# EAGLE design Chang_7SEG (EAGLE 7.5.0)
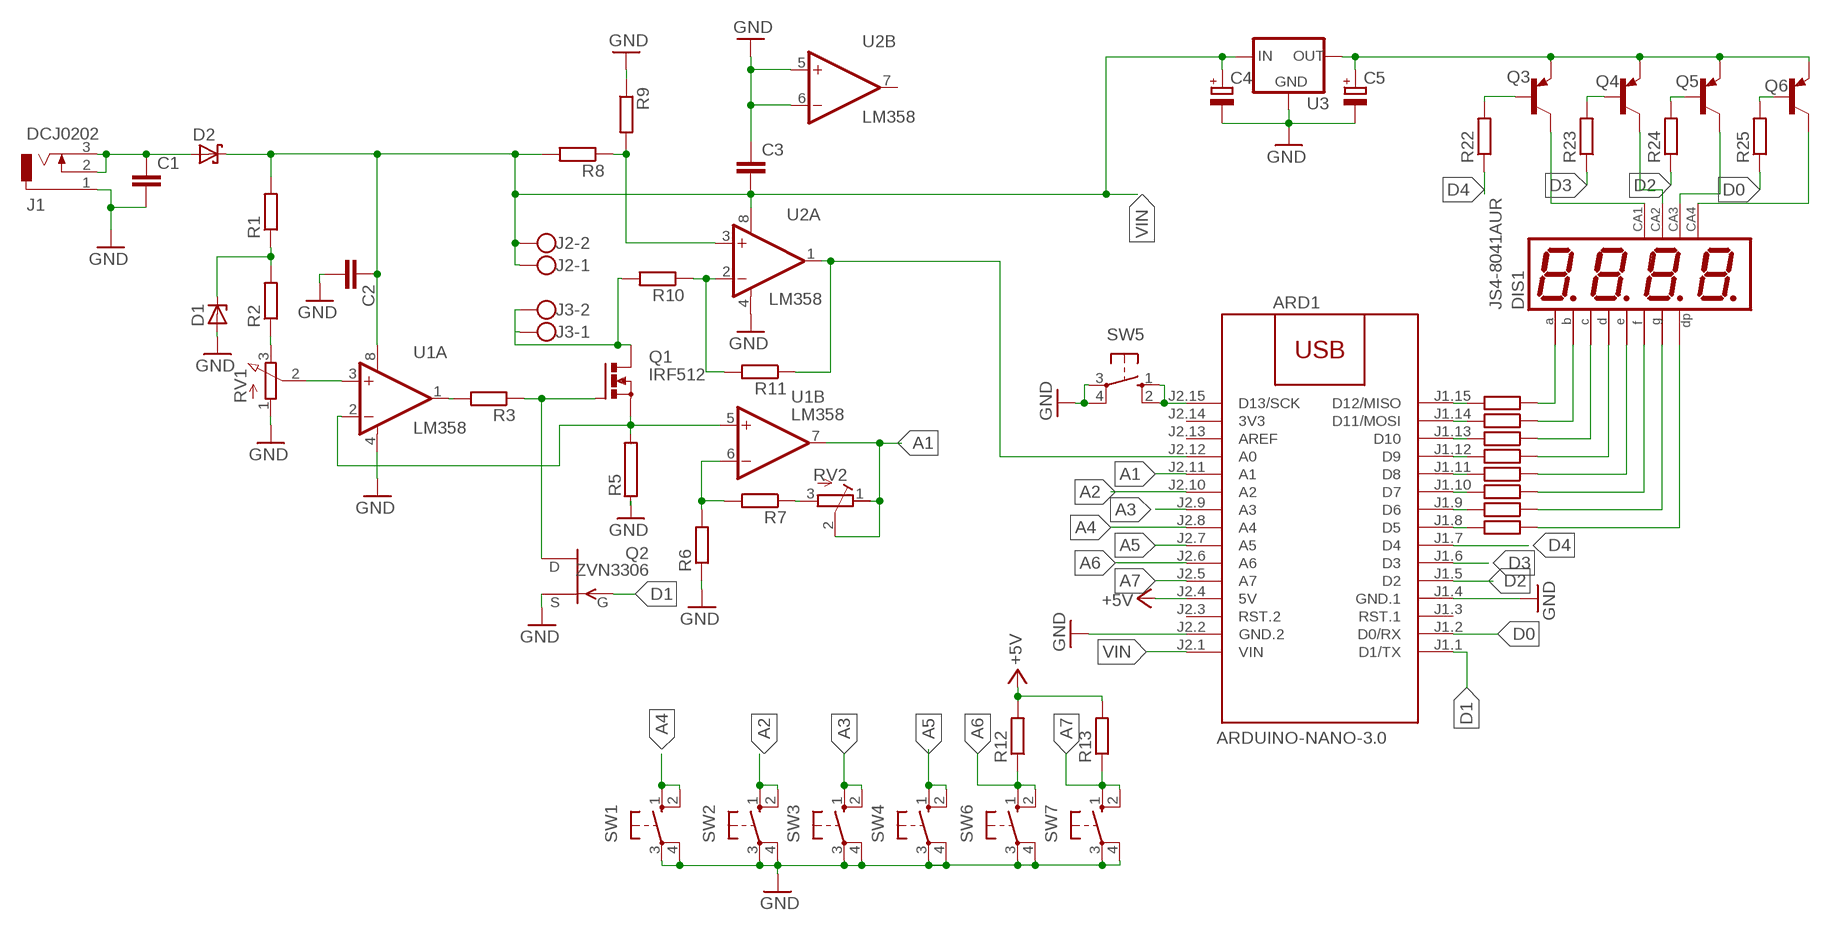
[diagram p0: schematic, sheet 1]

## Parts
ARD1  ARDUINO-NANO-3.0  [ARDUINO-NANO-3.0]
C1  C-EUC1206  [C1206]
C2  C-EUC1206  [C1206]
C3  C-EUC1206  [C1206]
C4  CPOL-EUSMCC  [SMC_C]
C5  CPOL-EUSMCC  [SMC_C]
D1  1N4728  [DO41Z10]
D2  MBR1560  [TO220ACS]
DIS1  JS4-8041AUR  [0.8INCH-4DIG]
J1  DCJ0202  [DCJ0202]
J2  W237-102  [W237-102]
J3  W237-102  [W237-102]
Q1  IRF512  [TO220BV]
Q2  ZVN3306  2N3819  [TO92]
Q3  BC328  [TO92-EBC]
Q4  BC328  [TO92-EBC]
Q5  BC328  [TO92-EBC]
Q6  BC328  [TO92-EBC]
R1  R-EU_R1206  [R1206]
R2  R-EU_R1206  [R1206]
R3  R-EU_R1206  [R1206]
R5  RAC04  [AC04]
R6  R-EU_R1206  [R1206]
R7  R-EU_R1206  [R1206]
R8  R-EU_R1206  [R1206]
R9  R-EU_R1206  [R1206]
R10  R-EU_R1206  [R1206]
R11  R-EU_R1206  [R1206]
R12  R-EU_R1206  [R1206]
R13  R-EU_R1206  [R1206]
R14  R-EU_R1206  [R1206]
R15  R-EU_R1206  [R1206]
R16  R-EU_R1206  [R1206]
R17  R-EU_R1206  [R1206]
R18  R-EU_R1206  [R1206]
R19  R-EU_R1206  [R1206]
R20  R-EU_R1206  [R1206]
R21  R-EU_R1206  [R1206]
R22  R-EU_R1206  [R1206]
R23  R-EU_R1206  [R1206]
R24  R-EU_R1206  [R1206]
R25  R-EU_R1206  [R1206]
RV1  PV09A  [PTV09]
RV2  R-TRIMM-3386-F  [R-TRIMM-3386F]
SW1  40-XX  [B3F-40XX]
SW2  40-XX  [B3F-40XX]
SW3  40-XX  [B3F-40XX]
SW4  40-XX  [B3F-40XX]
SW5  40-XX  [B3F-40XX]
SW6  40-XX  [B3F-40XX]
SW7  40-XX  [B3F-40XX]
U1  LM358  OPA2650P  [DIL08]
U2  LM358  OPA2650P  [DIL08]
U3  78XXS  [78XXS]

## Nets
+5V: ARD1.J2.4(5V) R12.2 R13.2
A1: ARD1.J2.11(A1) RV2.1(A) RV2.2(S) U1.7(B:OUT)
A2: ARD1.J2.10(A2) SW2.1(S) SW2.2(S1)
A3: ARD1.J2.9(A3) SW3.1(S) SW3.2(S1)
A4: ARD1.J2.8(A4) SW1.1(S) SW1.2(S1)
A5: ARD1.J2.7(A5) SW4.1(S) SW4.2(S1)
A6: ARD1.J2.6(A6) R12.1 SW6.1(S) SW6.2(S1)
A7: ARD1.J2.5(A7) R13.1 SW7.1(S) SW7.2(S1)
D0: ARD1.J1.2(D0/RX) R25.1
D1: ARD1.J1.1(D1/TX) Q2.2(G)
D2: ARD1.J1.5(D2) R24.1
D3: ARD1.J1.6(D3) R23.1
D4: ARD1.J1.7(D4) R22.1
GND: ARD1.J1.4(GND.1) ARD1.J2.2(GND.2) C1.2 C2.2 C3.1 C4.- C5.- D1.A J1.1 Q2.3(S) R5.1 R6.1 R9.1 RV1.1(A) SW1.3(P) SW1.4(P1) SW2.3(P) SW2.4(P1) SW3.3(P) SW3.4(P1) SW4.3(P) SW4.4(P1) SW5.3(P) SW5.4(P1) SW6.3(P) SW6.4(P1) SW7.3(P) SW7.4(P1) U1.4(A:V-) U2.4(A:V-) U2.5(B:+IN) U2.6(B:-IN) U3.GND
N$1: Q3.B R22.2
N$2: Q4.B R23.2
N$3: DIS1.12(CA) Q3.C
N$4: DIS1.9(CA) Q4.C
N$5: Q5.B R24.2
N$6: DIS1.8(CA) Q5.C
N$7: C1.1 D2.A J1.2 J1.3
N$8: Q6.B R25.2
N$9: DIS1.6(CA4) Q6.C
N$10: ARD1.J1.15(D12/MISO) R14.2
N$11: ARD1.J1.14(D11/MOSI) R15.2
N$12: ARD1.J1.13(D10) R16.2
N$13: ARD1.J1.12(D9) R17.2
N$14: ARD1.J1.11(D8) R18.2
N$15: ARD1.J1.10(D7) R19.2
N$16: ARD1.J1.9(D6) R20.2
N$17: ARD1.J1.8(D5) R21.2
N$18: DIS1.11(A) R14.1
N$19: DIS1.7(B) R15.1
N$20: DIS1.4(C) R16.1
N$21: DIS1.2(D) R17.1
N$22: DIS1.1(E) R18.1
N$23: DIS1.10(F) R19.1
N$24: DIS1.5(G) R20.1
N$25: DIS1.3(DP) R21.1
N$26: C5.+ Q3.E Q4.E Q5.E Q6.E U3.OUT
N$27: R2.1 RV1.3(E)
N$28: RV1.2(S) U1.3(A:+IN)
N$29: D1.C R1.1 R2.2
N$30: R3.2 U1.1(A:OUT)
N$31: ARD1.J2.15(D13/SCK) SW5.1(S) SW5.2(S1)
N$32: Q1.G Q2.1(D) R3.1
N$33: Q1.S R5.2 U1.2(A:-IN) U1.5(B:+IN)
N$34: J3.1 J3.2 Q1.D R10.2
N$35: R7.1 RV2.3(E)
N$36: R6.2 R7.2 U1.6(B:-IN)
N$37: R8.1 R9.2 U2.3(A:+IN)
N$38: R10.1 R11.2 U2.2(A:-IN)
N$39: ARD1.J2.12(A0) R11.1 U2.1(A:OUT)
VIN: ARD1.J2.1(VIN) C2.1 C3.2 C4.+ D2.C J2.1 J2.2 R1.2 R8.2 U1.8(A:V+) U2.8(A:V+) U3.IN
Unconnected: ARD1.J1.3(RST.1) ARD1.J2.3(RST.2) ARD1.J2.13(AREF) U2.7(B:OUT)

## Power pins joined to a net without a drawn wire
3V3: ARD1.J2.14(3V3)

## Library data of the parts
ARD1 = diy-modules:ARDUINO-NANO-3.0: Arduino Nano 3.0 and compatible devices More details available here: https://www.arduino.cc/en/Main/ArduinoBoardNano Click here to find device on ebay.com
C1-C3 = rcl:C-EU: CAPACITOR, European symbol
C4 C5 = rcl:CPOL-EU: POLARIZED CAPACITOR, European symbol
D1 = diode:1N4728: Z DIODE
D2 = diode:MBR1560
DIS1 = display-kingbright:JS4-8041AUR: 0.8in 4digit display CA
J1 = con-jack:DCJ0202: DC POWER JACK Source: DCJ0202.pdf; OC_FARNELL: unknown; OC_NEWARK: unknown
J2 J3 = con-wago-500:W237-102: WAGO SCREW CLAMP; MPN: 237-102; OC_FARNELL: unknown; OC_NEWARK: 70K9898
Q1 = transistor-power:IRF512: N-CHANNEL MOS FET
Q2 = transistor-fet:2N3819: N-Channel Junction FET
Q3-Q6 = transistor-pnp:BC328*: PNP Transistror
R1-R3 R6-R25 = rcl:R-EU_: RESISTOR, European symbol
R5 = resistor-power:R: Power Resitor; OC_FARNELL: unknown; OC_NEWARK: unknown
RV1 = pot:PV09A
RV2 = rcl:R-TRIMM-3386-F
SW1-SW7 = switch-omron:40-XX: OMRON SWITCH; MF: OMRON COMPONENTS USA; MPN: B3F-4000; OC_FARNELL: 176434; OC_NEWARK: 36K3105
U1 U2 = burr-brown:OPA2650: Dual Wideband, Low Power Voltage Feedback Operational Amplifier; MPN: AD8056ANZ; OC_FARNELL: 1079308; OC_NEWARK: 19M0925
U3 = v-reg:78XXS: VOLTAGE REGULATOR

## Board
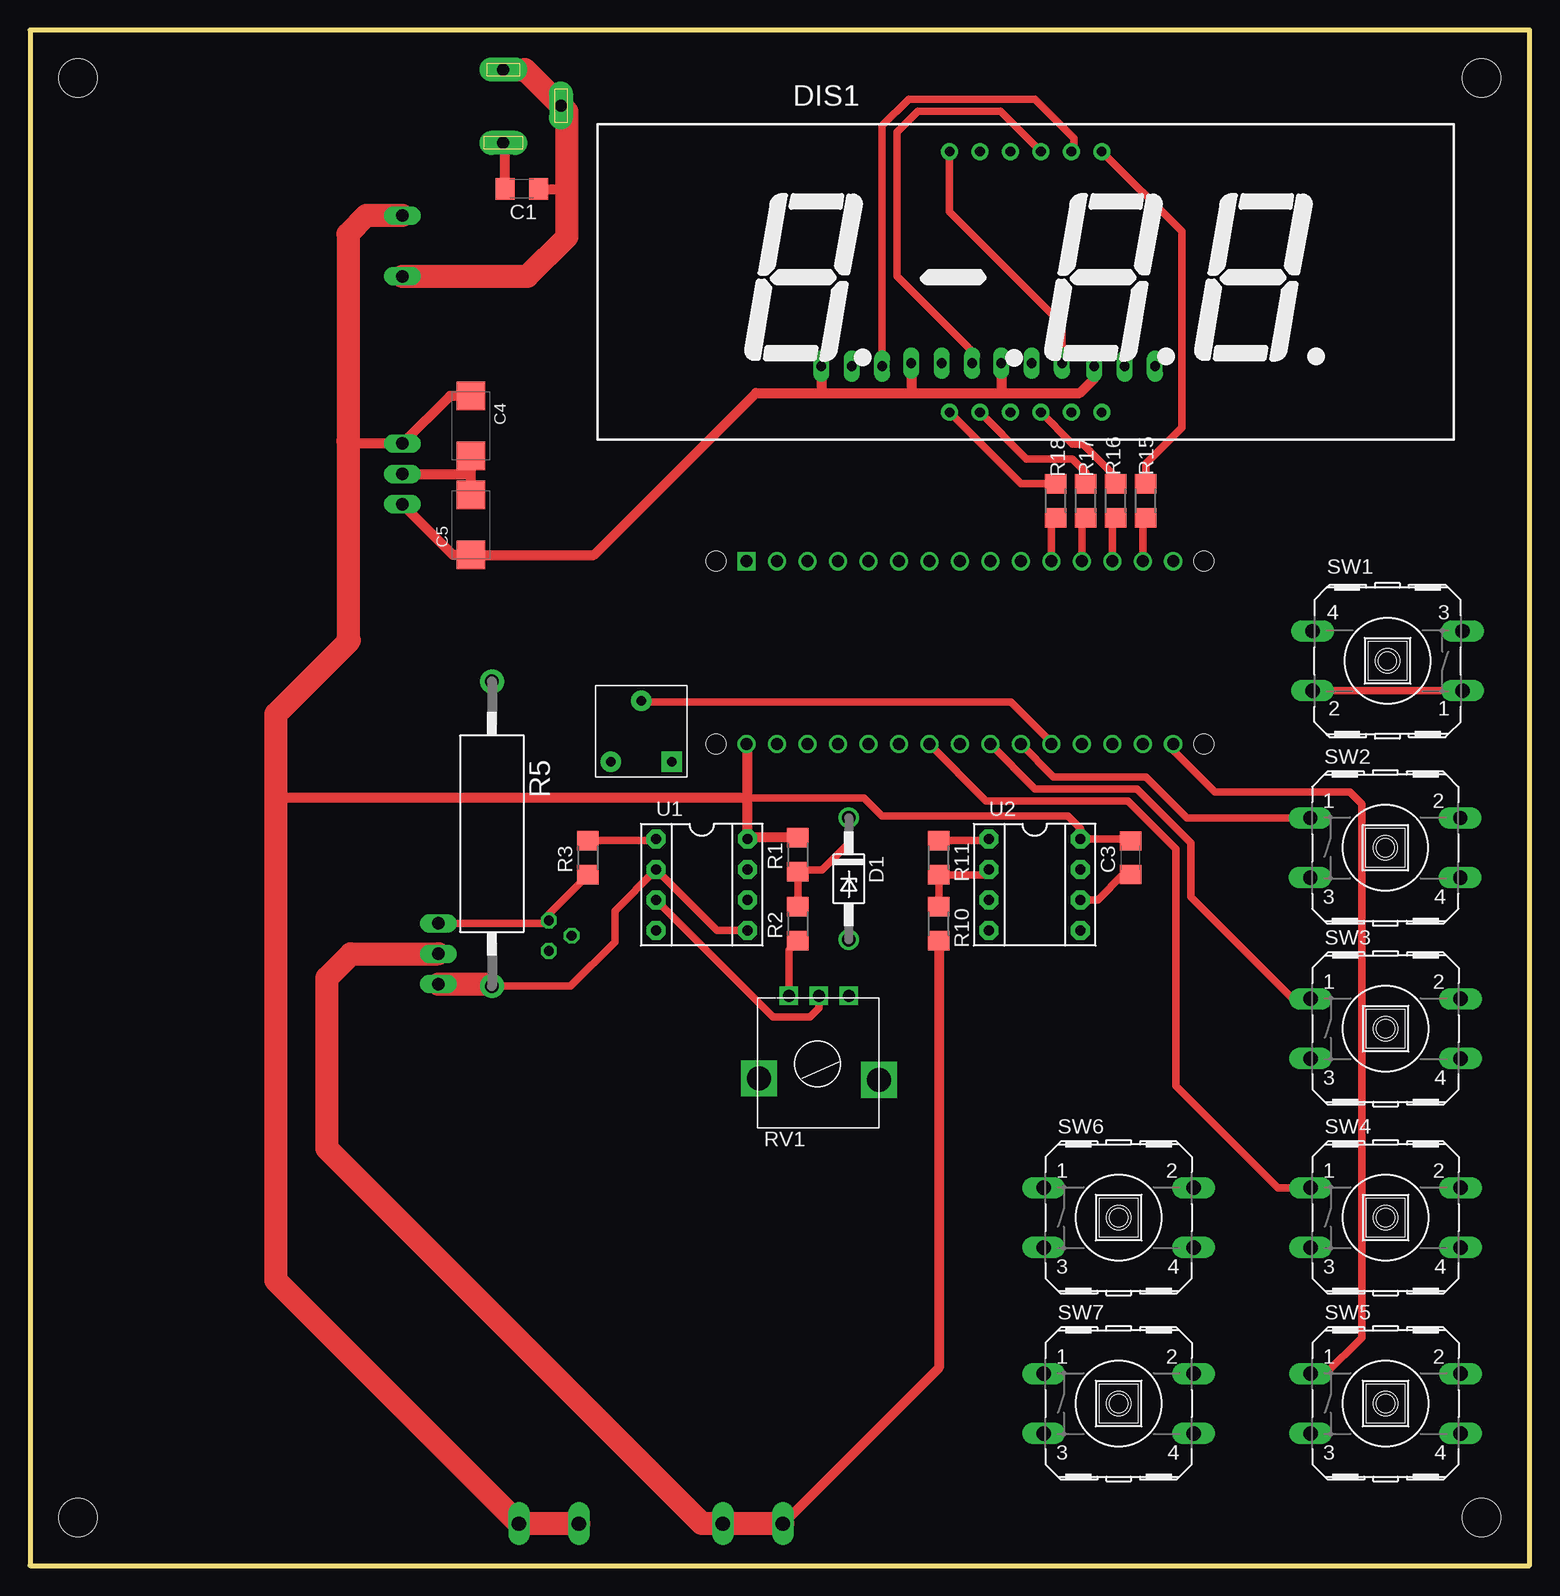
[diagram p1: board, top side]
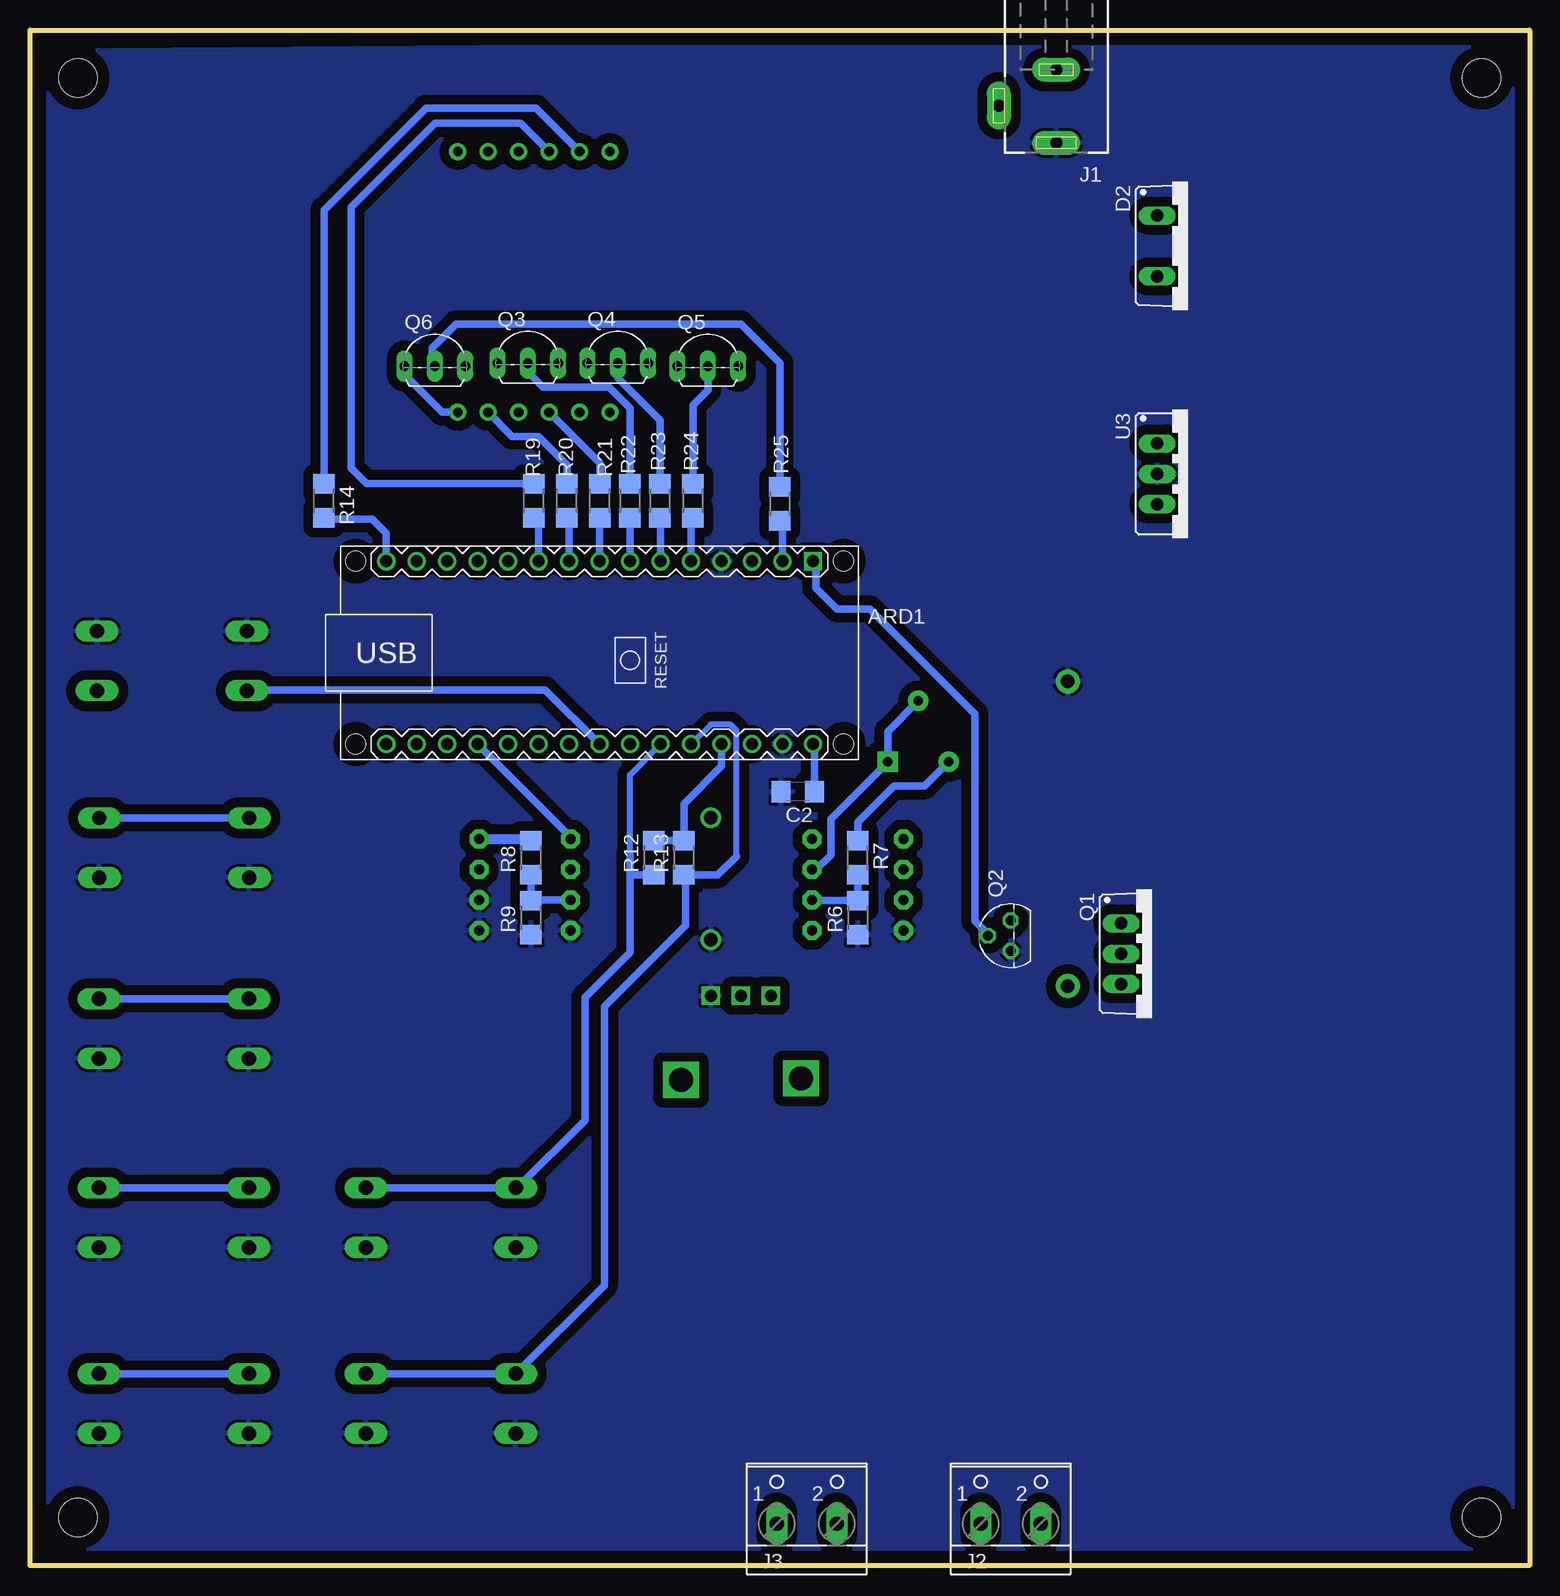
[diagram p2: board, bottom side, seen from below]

Size 125 x 128 mm. Coordinates in mm from the lower left corner, seen from the top.
Outline: 0,0 125,0 125,128 0,128 0,0
Copper layers (1*16): Top 0.035mm / dielectric 1.5mm / Bottom 0.035mm
Design rules "default": minimum track width 10mil, minimum drill 24mil, track to track 8mil, track to pad 8mil, pad to pad 8mil, via to via 8mil, smd to smd 8mil, copper to edge 40mil, drill to drill 8mil, minimum pad ring 10mil, minimum via ring 8mil, stop-mask expansion 4mil, vias tented up to drill 0mil, thermal gap 10mil
Holes 3.2 mm at 4,4 121,4 4,124 121,124

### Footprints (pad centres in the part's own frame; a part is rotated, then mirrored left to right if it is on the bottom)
ARDUINO-NANO-3.0 = drill 1 square: J1.1 17.78,7.62 | drill 1: J1.2 15.24,7.62; J1.3 12.7,7.62; J1.4 10.16,7.62; J1.5 7.62,7.62; J1.6 5.08,7.62; J1.7 2.54,7.62; J1.8 0,7.62; J1.9 -2.54,7.62; J1.10 -5.08,7.62; J1.11 -7.62,7.62; J1.12 -10.16,7.62; J1.13 -12.7,7.62; J1.14 -15.24,7.62; J1.15 -17.78,7.62; J2.1 17.78,-7.62; J2.2 15.24,-7.62; J2.3 12.7,-7.62; J2.4 10.16,-7.62; J2.5 7.62,-7.62; J2.6 5.08,-7.62; J2.7 2.54,-7.62; J2.8 0,-7.62; J2.9 -2.54,-7.62; J2.10 -5.08,-7.62; J2.11 -7.62,-7.62; J2.12 -10.16,-7.62; J2.13 -12.7,-7.62; J2.14 -15.24,-7.62; J2.15 -17.78,-7.62 | hole 1.651: -20.32,7.62; -20.32,-7.62; 20.32,-7.62; 20.32,7.62
C1206 = smd 1.6 x 1.8: 1 -1.4,0; 2 1.4,0
SMC_C = smd 2.4 x 2.4: + -2.5,0; - 2.5,0
DO41Z10 = drill 1.118: A 5.08,0; C -5.08,0
TO220ACS = drill 1.016 long: A 2.54,-2.54; C -2.54,-2.54
0.8INCH-4DIG = drill 0.8 pad 1.422: 1 29.15,2.38; 2 31.69,2.38; 3 34.23,2.38; 4 36.77,2.38; 5 39.31,2.38; 6 41.85,2.38; 7 41.85,24.12; 8 39.31,24.12; 9 36.77,24.12; 10 34.23,24.12; 11 31.69,24.12; 12 29.15,24.12
DCJ0202 = drill 1 pad 2 long: 1 0,3.1; 2 4.8,0; 3 0,-3
W237-102 = drill 1.194 long: 1 -2.5,-1.27; 2 2.5,-1.27
TO220BV = drill 1.016 long: D 0,-2.54; G -2.54,-2.54; S 2.54,-2.54
TO92 = drill 0.813 octagon: 1 1.27,0; 2 0,1.905; 3 -1.27,0
TO92-EBC = drill 0.813 long: B 0,-1.27; C -2.54,-1.27; E 2.54,-1.27
R1206 = smd 1.6 x 1.803: 1 -1.422,0; 2 1.422,0
AC04 = drill 1.1 pad 2: 1 -12.7,0; 2 12.7,0
PTV09 = drill 1 square: 1 -2.5,0; 2 0,0; 3 2.5,0 | drill 2 square: P$4 -5,7; P$5 5,6.9
R-TRIMM-3386F = drill 0.8 pad 1.676 square: 1 0,0 | drill 0.8 pad 1.676: 2 5.08,2.54; 3 0,5.08
B3F-40XX = drill 1.194 long: 1 -6.248,2.489; 2 6.248,2.489; 3 -6.248,-2.489; 4 6.248,-2.489
DIL08 = drill 0.813 pad 1.6 octagon: 1 -3.81,-3.81; 2 -1.27,-3.81; 3 1.27,-3.81; 4 3.81,-3.81; 5 3.81,3.81; 6 1.27,3.81; 7 -1.27,3.81; 8 -3.81,3.81
78XXS = drill 1.016 long: GND 0,-2.54; IN -2.54,-2.54; OUT 2.54,-2.54

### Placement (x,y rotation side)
ARD1  77.52,76.09 0 bottom
C1  41,114.75 180 top
C2  61,64.5 180 bottom
C3  91.75,59 90 top
C4  36.75,95 270 top
C5  36.75,86.75 90 top
D1  68.25,57.25 270 top
D2  28.5,110 270 bottom
DIS1  47.5,93.75 0 top
J1  39.45,121.69 180 bottom
J2  43.25,4.75 0 bottom
J3  60.25,4.75 0 bottom
Q1  31.5,51 270 bottom
Q2  43.25,52.5 90 bottom
Q3  83.5,101.5 0 bottom
Q4  76,101.5 0 bottom
Q5  68.5,101.25 0 bottom
Q6  91.25,101.25 0 bottom
R1  64,59.25 90 top
R2  64,53.5 90 top
R3  46.5,59 90 top
R5  38.5,61 270 top
R6  56,54 90 bottom
R7  56,59 270 bottom
R8  83.25,59 90 bottom
R9  83.25,54 90 bottom
R10  75.75,53.5 270 top
R11  75.75,59 270 top
R12  73,59 90 bottom
R13  70.5,59 90 bottom
R14  100.5,88.75 270 bottom
R15  93,88.75 270 top
R16  90.5,88.75 270 top
R17  88,88.75 270 top
R18  85.5,88.75 270 top
R19  83,88.75 270 bottom
R20  80.25,88.75 270 bottom
R21  77.5,88.75 270 bottom
R22  75,88.75 90 bottom
R23  72.5,88.75 90 bottom
R24  69.75,88.75 90 bottom
R25  62.5,88.5 90 bottom
RV1  65.75,47.5 180 top
RV2  53.5,67 90 top
SW1  113.16,75.41 180 top
SW2  112.97,59.83 0 top
SW3  113,44.75 0 top
SW4  113,29 0 top
SW5  113,13.5 0 top
SW6  90.75,29 0 top
SW7  90.75,13.5 0 top
U1  56,56.75 270 top
U2  83.75,56.75 270 top
U3  28.5,91 270 bottom

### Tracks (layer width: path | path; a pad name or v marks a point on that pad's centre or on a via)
+5V
  Bottom 0.61: ARD1.J2.4 67.36,66.65 70.5,63.5 R13.2 R12.2
A1
  Top 0.61: ARD1.J2.11 85.14,68.62 81.75,72 51.04,72 RV2.2
  Bottom 0.61: U1.7 59.48,58.02 58.25,59.25 58.25,62.25 RV2.1 53.5,69.54 RV2.2 51.13,72.25
A2
  Top 0.61: SW2.1 96.43,62.32 93,65.75 85.31,65.75 ARD1.J2.10
  Bottom 0.61: SW2.1 SW2.2
A3
  Top 0.61: SW3.1 105.26,47.24 96.75,55.75 96.75,60.25 92.25,64.75 83.78,64.75 ARD1.J2.9
  Bottom 0.61: SW3.1 SW3.2
A4
  Top 0.61: SW1.2 106.83,73 106.25,73 106.33,72.92 SW1.1
  Bottom 0.61: ARD1.J2.8 82.05,73 106.83,73 SW1.2
A5
  Top 0.61: SW4.1 104.01,31.49 95.5,40 95.5,59.75 91.5,63.75 79.69,63.75 ARD1.J2.7
  Bottom 0.61: SW4.1 SW4.2
A6
  Bottom 0.5: 75,58.5 75,59.25 75,65.91 ARD1.J2.6
  Bottom 0.61: 75,57.38 75,51.12 78.75,47.38 78.75,37.12 84.39,31.49 SW6.1 SW6.2 | 75,57.38 75,59.25 | R12.1 74.8,57.58 75,57.38
A7
  Bottom 0.5: 66.12,59.12 66.12,69.62 66.62,70.12 68.24,70.12 ARD1.J2.5
  Bottom 0.61: 66.12,59.12 67.67,57.58 R13.1 70.38,57.45 70.38,53.38 77.12,46.62 77.12,23.37 SW7.1 SW7.2
D0
  Bottom 0.61: ARD1.J1.2 62.27,86.85 R25.1
D1
  Bottom 0.61: Q2.2 45.16,52.66 46.25,53.75 46.25,71 55,79.75 57.75,79.75 59.5,81.5 59.5,83.47 ARD1.J1.1
D2
  Bottom 0.61: ARD1.J1.5 69.89,87.18 R24.1
D3
  Bottom 0.61: ARD1.J1.6 72.44,87.26 R23.1
D4
  Bottom 0.61: ARD1.J1.7 74.97,87.3 R22.1
GND
  Top 0.61: C3.1 91.1,57.6 89,55.5 87.58,55.5 U2.6
  Top 0.813: C5.- 36.75,90.75 | 36.75,90.75 C4.- | U3.GND 36.5,91 36.75,90.75 | C1.2 39.6,118.44 J1.1
  pour Bottom (isolate 0.813): 1,127.25 123.5,126.25 123.5,-0.5 1,0.5
N$1
  Bottom 0.61: R22.2 75,96.5 76.75,98.25 82.25,98.25 83.5,99.5 Q3.B
N$2
  Bottom 0.61: R23.2 72.5,95.5 76,99 Q4.B
N$3
  Top 0.61: DIS1.12 76.65,112.85 86,103.5 86,100.27 Q3.C
N$4
  Top 0.61: Q4.C 78.54,101.21 72.25,107.5 72.25,119.5 74,121.25 80.89,121.25 DIS1.9
N$5
  Bottom 0.61: R24.2 69.75,96.75 68.5,98 Q5.B
N$6
  Top 0.61: Q5.C 71.04,120.04 73.25,122.25 83.75,122.25 87,119 87,118.06 DIS1.8
N$7
  Top 0.813: C1.1 44.5,114.75 44.75,115
  Top 1.93: D2.A 41.46,107.46 44.75,110.75 44.75,115 44.75,121.19 J1.2 41.25,124.69 J1.3
N$8
  Bottom 0.61: R25.2 62.5,100.25 65.75,103.5 89.5,103.5 91.5,101.5 91.5,100.23 Q6.B
N$9
  Bottom 0.61: DIS1.6 90.63,96.13 93.75,99.25 93.75,99.94 Q6.C
N$10
  Bottom 0.61: ARD1.J1.15 95.3,86.05 96.5,87.25 100.58,87.25 | 101,87.25 100.58,87.25 | 100.58,87.25 R14.2
N$11
  Top 0.61: ARD1.J1.14 92.75,87.08 R15.2
N$12
  Top 0.61: ARD1.J1.13 90.22,87.04 R16.2
N$13
  Top 0.61: ARD1.J1.12 87.67,87 R17.2
N$14
  Top 0.61: ARD1.J1.11 85.14,86.96 R18.2
N$15
  Bottom 0.61: ARD1.J1.10 82.59,86.92 R19.2
N$16
  Bottom 0.61: ARD1.J1.9 80.06,87.13 R20.2
N$17
  Bottom 0.61: ARD1.J1.8 77.52,87.31 R21.2
N$18
  Bottom 0.61: R14.1 100.5,113 92,121.5 82.82,121.5 DIS1.11
N$19
  Top 0.61: R15.1 93,91.88 96,94.88 96,111.22 DIS1.7
N$20
  Top 0.61: R16.1 90.5,90.75 87.75,93.5 86.9,93.5 DIS1.4
N$21
  Top 0.61: R17.1 88,91.12 86.88,92.25 83.07,92.25 DIS1.2
N$22
  Top 0.61: R18.1 82.61,90.17 DIS1.1
N$23
  Bottom 0.61: R19.1 96.92,90.17 98.25,91.5 98.25,113.25 91.25,120.25 84.11,120.25 DIS1.10
N$24
  Bottom 0.61: R20.1 80.25,91.75 82.62,94.12 84.81,94.12 DIS1.5
N$25
  Bottom 0.61: R21.1 77.5,91.9 DIS1.3
N$26
  Top 0.813: Q5.E 65.96,97.96 65.75,97.75 | 73.25,97.75 80.75,97.75 | 80.75,97.75 87.5,97.75 88.75,99 88.75,99.94 Q6.E | Q3.E 80.96,97.96 80.75,97.75 | Q4.E 73.46,97.96 73.25,97.75 | 65.75,97.75 60.5,97.75 47,84.25 C5.+ 35.25,84.25 U3.OUT | 65.75,97.75 73.25,97.75
N$27
  Top 0.61: RV1.3 63.25,51.33 R2.1
N$28
  Top 0.61: RV1.2 65.75,46.5 65,45.75 61.92,45.75 U1.3
N$29
  Top 0.61: R2.2 R1.1 64.17,58 66,58 68.25,60.25 D1.C
N$30
  Top 0.61: R3.2 52.05,60.42 U1.1
N$31
  Top 0.61: SW5.1 107.99,15.99 111,19 111,63.5 110,64.5 98.75,64.5 95.3,67.95 ARD1.J2.15
  Bottom 0.61: SW5.2 SW5.1
N$32
  Top 0.61: R3.1 43.25,54.33 Q2.1 43.02,53.54 Q1.G
N$33
  Top 0.61: U1.5 57.27,52.94 U1.2 48.75,54.58 48.75,52 45.05,48.3 R5.2
  Top 1.93: Q1.S 38.34,48.46 R5.2
N$34
  Top 0.813: R10.2 75.75,16.48 J3.1
  Top 1.93: Q1.D 26.75,51 24.75,49 24.75,34.75 56.02,3.48 J3.2 J3.1
N$35
  Bottom 0.61: R7.1 56,62 53,65 50.42,65 RV2.3
N$36
  Bottom 0.61: R7.2 R6.2 59.75,55.42 U1.6
N$37
  Bottom 0.61: R8.1 R9.2 83.19,55.48 U2.3
N$38
  Top 0.61: U2.2 79.5,57.58 R11.2 R10.1
N$39
  Top 0.61: R11.1 79.8,60.42 U2.1
  Bottom 0.61: U2.1 79.94,60.73 ARD1.J2.12
VIN
  Top 0.61: U2.8 91.59,60.56 C3.2 | 87.56,61.19 87.56,61.44 86.5,62.5 71,62.5 69.5,64 59.81,64
  Top 0.813: 26.5,93.75 26.71,93.54 U3.IN 35,97.5 C4.+ | 27,76.75 26.62,77.12 26.5,77.25 | 59.81,64 U1.8 59.92,60.67 R1.2 | U2.8 87.56,61.19 | 59.81,64 20.75,64 20.5,63.75 | 59.81,64 59.81,68.4 ARD1.J2.1
  Top 1.93: D2.C 28.04,112.54 26.5,111 26.5,93.75 26.5,77.25 | 26.62,77.12 20.5,71 20.5,63.75 20.5,23.75 40.75,3.5 J2.2 J2.1
  Bottom 0.61: C2.1 59.6,68.34 ARD1.J2.1
  Bottom 0.813: U2.8 83.39,60.56 R8.2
